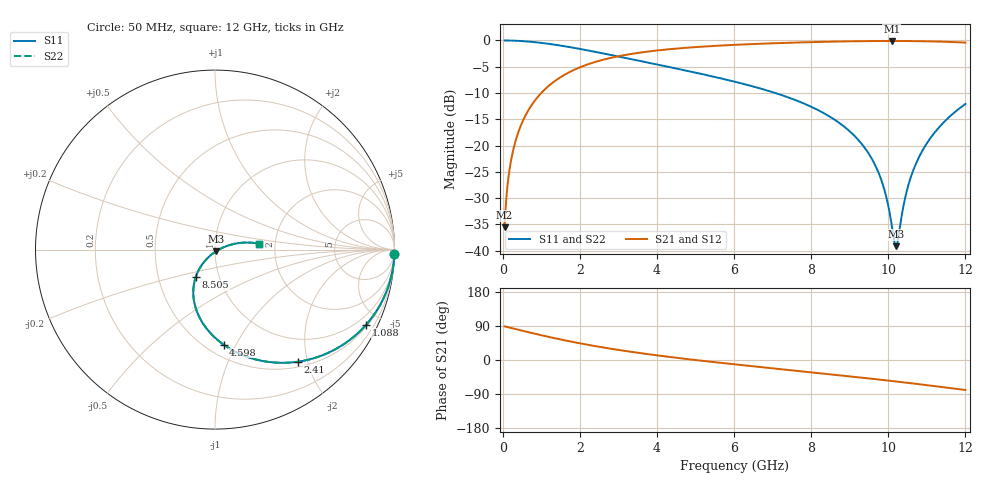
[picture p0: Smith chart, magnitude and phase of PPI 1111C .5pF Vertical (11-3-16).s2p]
# GHz S MA R 50
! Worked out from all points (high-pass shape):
!   1601 points, 50 MHz to 12 GHz, reference 50 ohm
!   highest |S21| = -0.10 dB at 10.09 GHz (marker M1); lowest = -35.6 dB at 50 MHz (marker M2)
!   |S21| within 3 dB of the highest: 2.937 GHz to end of sweep
!   lowest |S11| = -39.1 dB at 10.2 GHz (marker M3), VSWR 1.02, Z = 50.6 - j0.943 ohm
!   |S11| at or under -10 dB: 7.072 GHz to end of sweep
!   |S22| runs from -39.1 to 0.0 dB; largest |S21 - S12| = 0
!   S11 on the Smith chart (normalised r, x): 50 MHz: 1, -91; 1.088 GHz: 0.58, -4.16; 2.41 GHz: 0.58, -1.84; 4.598 GHz: 0.60, -0.89; 8.505 GHz: 0.77, -0.24; 12 GHz: 1.65, +0.12
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0.05  0.9999 -1.3  0.01668 88.7  0.01668 88.7  0.9999 -1.3
0.1919063  0.9979 -4.8  0.06391 85.2  0.06391 85.2  0.9979 -4.8
0.3711563  0.9924 -9.3  0.1229 80.7  0.1229 80.7  0.9924 -9.3
0.6699063  0.9758 -16.7  0.2181 73.3  0.2181 73.3  0.9758 -16.7
1.088156  0.9397 -26.6  0.3411 63.4  0.3411 63.4  0.9397 -26.6
2.044156  0.8252 -46.7  0.563 43.2  0.563 43.2  0.8252 -46.7
2.410125  0.7778 -53.4  0.6262 36.5  0.6262 36.5  0.7778 -53.4
4.038312  0.5872 -77.9  0.8056 11.8  0.8056 11.8  0.5872 -77.9
4.598469  0.5315 -84.9  0.8426 4.7  0.8426 4.7  0.5315 -84.9
6.025  0.4047 -100.8  0.9086 -11.5  0.9086 -11.5  0.4047 -100.8
8.019156  0.2325 -120.6  0.9644 -32.5  0.9644 -32.5  0.2325 -120.6
8.504625  0.1866 -125.1  0.9736 -37.7  0.9736 -37.7  0.1866 -125.1
9.497969  0.08335 -131.8  0.9862 -48.6  0.9862 -48.6  0.08335 -131.8
9.804187  0.04887 -129.8  0.988 -52.1  0.988 -52.1  0.04887 -129.8
10.01331  0.02533 -119.4  0.9885 -54.5  0.9885 -54.5  0.02533 -119.4
10.088  0.01764 -107.3  0.9885 -55.3  0.9885 -55.3  0.01764 -107.3
10.20003  0.01106 -57.4  0.9884 -56.7  0.9884 -56.7  0.01106 -57.4
10.25231  0.01283 -27.6  0.9883 -57.3  0.9883 -57.3  0.01283 -27.6
10.50625  0.04026 13.0  0.9872 -60.3  0.9872 -60.3  0.04026 13.0
10.805  0.07881 17.2  0.9843 -63.9  0.9843 -63.9  0.07881 17.2
11.31288  0.1486 14.7  0.9754 -70.3  0.9754 -70.3  0.1486 14.7
12  0.2491 7.6  0.9537 -79.2  0.9537 -79.2  0.2491 7.6
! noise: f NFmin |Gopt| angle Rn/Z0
0.05  0.001679  0.9835  1.216  0.02319
1.372  0.005861  0.7925  12.01  0.005765
2.701  0.009523  0.747  19.14  0.007366
4.031  0.0129  0.7268  26.34  0.008915
5.36  0.0162  0.7185  33.4  0.01048
6.682  0.01954  0.7181  40.17  0.01214
8.012  0.02305  0.7234  46.68  0.01401
9.341  0.02683  0.7333  52.85  0.0162
10.67  0.031  0.7469  58.69  0.01884
12  0.03571  0.7632  64.2  0.02213
